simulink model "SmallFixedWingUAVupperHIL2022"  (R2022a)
settings: Solver=FixedStepDiscrete  StartTime=0.0  StopTime=inf  FixedStep=1/150  RelTol=1e-3
model workspace: external: MAT-File (data not in the file)
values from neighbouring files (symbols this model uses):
  env = struct    [InitDatactrl.m]
  uav = struct    [InitDatactrl.m]    (also in InitDatactrldf.m)
  x = x + points(1, i) * k(i) * ft    [bezir_n.m]
undefined symbols (not defined in the file or in its folder): current_a, current_filtered_a, DiscIntNeverNeededParam, remaining, RGBLED_COLOR_ENUM, RGBLED_MODE_ENUM, voltage_filtered_v, voltage_v
libraries: simulink x10, pixhawk_slib_sensors_actuators x6, pixhawk_slib_uORB_RW x5

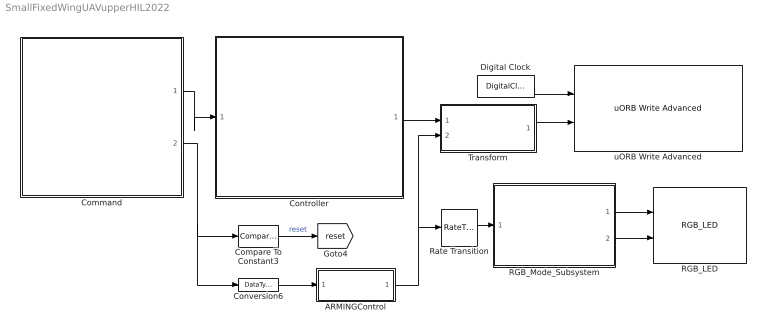
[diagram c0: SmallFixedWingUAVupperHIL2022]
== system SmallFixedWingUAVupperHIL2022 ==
  ARMINGControl : Subsystem
  Command : Subsystem
  Compare To Constant3 : simulink/Logic and Bit Operations/Compare To Constant  relop=<=  const=1100  OutDataTypeStr=boolean
  Controller : Subsystem
  Conversion6 : DataTypeConversion  OutDataTypeStr=double
  Digital Clock : DigitalClock  SampleTime=-1
  RGB_LED : pixhawk_slib_sensors_actuators/RGB_LED
  RGB_Mode_Subsystem : Subsystem
  Rate Transition : RateTransition  OutPortSampleTime=1
  Transform : Subsystem
  uORB Write Advanced : pixhawk_slib_uORB_RW/uORB Write Advanced  Ts=0  uORB_AdvtQueue=on  uORB_FieldEnabledArr="0  0  0  1  0  0  0  0  0  0  0"  uORB_Topic_str=0  uORB_Struct_DT="[1  1  1  1  1]"  BlockInputCount=5  uORB_StructParams="[\"voltage_v\",\"voltage_filtered_v\",\"current_a\",\"current_filtered_a\",\"remaining\"]"  uORB_PortSizes="[1  1  1  1]"  MsgSizeOf=0  MW_update=true
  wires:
  Digital Clock/1 -> uORB Write Advanced/1
  RGB_Mode_Subsystem/1(RGB_MODE) -> RGB_LED/1
  Rate Transition/1 -> RGB_Mode_Subsystem/1(ARM_STATE)
  ARMINGControl/1(Out1) -> Transform/2(Arm), Rate Transition/1
  RGB_Mode_Subsystem/2(RGB_COLOR) -> RGB_LED/2
  Conversion6/1 -> ARMINGControl/1(In1)
  Compare To Constant3/1 -> [reset]  "reset"
  Transform/1(PWMOuput) -> uORB Write Advanced/2
  Controller/1(ActuatorCmd) -> Transform/1(ActuatorCmd)
  Command/2(Arm) -> Conversion6/1, Compare To Constant3/1
  Command/1(Command) -> Controller/1(Cmd)

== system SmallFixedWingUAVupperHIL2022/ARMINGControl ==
  In1 : Inport
  Compare To Constant3 : simulink/Logic and Bit Operations/Compare To Constant  relop=>=  const=uint16(1500)  OutDataTypeStr=boolean
  Out1 : Outport  VectorParamsAs1DForOutWhenUnconnected=off
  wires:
  Compare To Constant3/1 -> Out1/1
  In1/1 -> Compare To Constant3/1

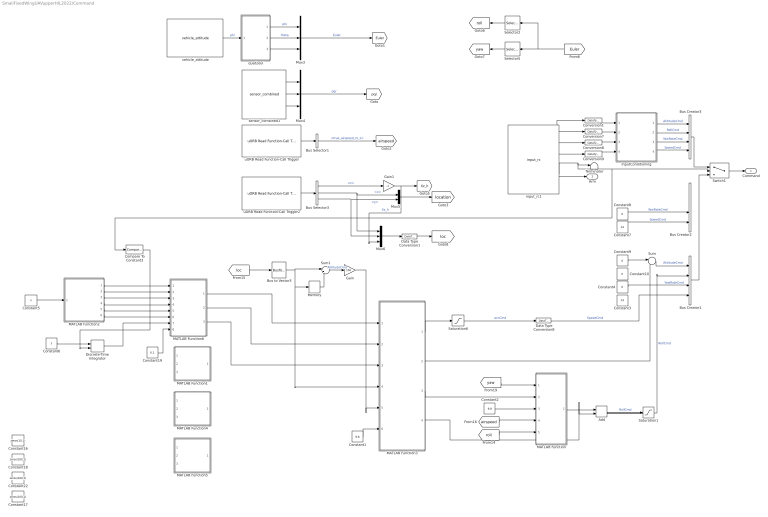
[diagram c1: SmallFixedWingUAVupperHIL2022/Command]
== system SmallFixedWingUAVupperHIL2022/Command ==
  Add : Sum
  Bus Creator1 : BusCreator  Inputs=4
  Bus Creator2 : BusCreator  Inputs=4
  Bus Creator3 : BusCreator  Inputs=4
  Bus Selector1 : BusSelector  OutputSignals=true_airspeed_m_s
  Bus Selector3 : BusSelector  OutputSignals=z,x,y
  Bus to Vector3 : BusToVector
  Compare To Constant3 : simulink/Logic and Bit Operations/Compare To Constant  relop=>=  const=uint16(1500)  OutDataTypeStr=boolean
  Constant1 : Constant  Value=9.8
  Constant{4,8..10} (4 alike) : Constant  Value=0  SampleTime=-1
  Constant16 : Constant  Value=zeros(10,1)
  Constant17 : Constant  Value=zeros(100,1)
  Constant18 : Constant  Value=zeros(100,1)
  Constant19 : Constant  Value=0.1
  Constant2 : Constant  Value=9.8  SampleTime=-1
  Constant22 : Constant  Value=zeros(100,1)
  Constant3 : Constant  Value=14  SampleTime=-1
  Constant5 : Constant  Value=x
  Constant6 : Constant
  Constant7 : Constant  Value=14  SampleTime=-1
  Conversion{1,7..9} (4 alike) : DataTypeConversion  OutDataTypeStr=double
  Data Type Conversion1 : DataTypeConversion  OutDataTypeStr=double
  Data Type Conversion8 : DataTypeConversion  OutDataTypeStr=single
  Discrete-Time Integrator : DiscreteIntegrator  ExternalReset=either  SampleTime=-1  ICPrevOutput=DiscIntNeverNeededParam  ICPrevScaledInput=DiscIntNeverNeededParam
  Gain : Gain  Gain=150
  Gain1 : Gain  Gain=-1
  InputConditioning : Subsystem
  MATLAB Function : MATLAB Function  TreatAsAtomicUnit=on
  MATLAB Function1 : MATLAB Function  Commented=on  TreatAsAtomicUnit=on
  MATLAB Function2 : MATLAB Function  TreatAsAtomicUnit=on
  MATLAB Function3 : MATLAB Function  TreatAsAtomicUnit=on
  MATLAB Function4 : MATLAB Function  Commented=on  TreatAsAtomicUnit=on
  MATLAB Function5 : MATLAB Function  Commented=on  TreatAsAtomicUnit=on
  MATLAB Function6 : MATLAB Function  TreatAsAtomicUnit=on
  Memory : Memory  InheritSampleTime=on
  Mux3 : Mux  Inputs=3
  Mux4 : Mux  Inputs=3
  Mux5 : Mux  Inputs=2
  Mux6 : Mux  Inputs=3
  Saturation1 : Saturate  UpperLimit=0.4  LowerLimit=-0.4
  Saturation6 : Saturate  UpperLimit=10  LowerLimit=-10
  Selector2 : Selector  InputPortWidth=3  IndexOptions=Index vector (dialog)  Indices=1  OutputSizes=1
  Selector5 : Selector  InputPortWidth=3  IndexOptions=Index vector (dialog)  Indices=3  OutputSizes=1
  Sum : Sum  Inputs=|++
  Sum1 : Sum  Inputs=|+-
  Switch1 : Switch  Criteria=u2 > Threshold  Threshold=1500
  Terminator : Terminator
  input_rc1 : pixhawk_slib_sensors_actuators/input_rc  Description=|  sampletime=1/150  channel1=on  channel2=on  channel3=on  channel4=on  channel5=on  channel6=on  channel7=off  channel8=off  channel9=off  channel10=off  channel11=off  channel12=off  channel13=off  channel14=off  channel15=off  channel16=off  channel17=off  channel18=off  ch_count=off  rssi=off  rc_failsafe=off  rc_lost=off  rc_inputsource=off
      | RC Input Block
      | 
      | This block provides user input control to the model.
      | It uses the input_rc uORB topic.
      | 
      | The user has the ability to choose which channels are available as outputs from this block and also some optional outputs. These include 
      | Channels 1 through 18
      | double data type indicating the PWM value from the controller 
      | measured pulse widths for each of the supported channels 
      | Channel Count 
      | u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
  quat2eul : MATLAB Function  TreatAsAtomicUnit=on
  sensor_combined1 : pixhawk_slib_sensors_actuators/sensor_combined  Description=|  sampletime=1/150  show_mag=off  show_acc=off  show_gyro=on  show_baro=off  show_ts=off
      | Sensor Combined Block
      | 
      | This block enables access to the various sensors available on the px4fmu-v2 hardware.  
      | The user can use these signals in the Simulink control model.  
      | The sample time needs to be provided in the mask dialog.  
      | Optional output ports can also be selected.  
      | Refer to the sample model: px4demo_attitude_control.slx
      | 
      | Signal definitions: 
      | Magnetometer (x,y,z) - single values – Mag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
  uORB Read Function-Call Trigger : pixhawk_slib_uORB_RW/uORB Read Function-Call Trigger  uORB_Topic_str='airspeed'  BusObjVar=Bus: airspeed_SL  uORB_Interval=1  AsyncOutput=off  Fcn_call_select=Generate Function Call Signal  TaskName='Task1'  Poll_timeout=100  Ts=-1
  uORB Read Function-Call Trigger2 : pixhawk_slib_uORB_RW/uORB Read Function-Call Trigger  uORB_Topic_str='vehicle_local_position'  BusObjVar=Bus: vehicle_local_position_SL  uORB_Interval=1  AsyncOutput=off  Fcn_call_select=Generate Function Call Signal  TaskName='Task1'  Poll_timeout=100  Ts=-1
  vehicle_attitude : pixhawk_slib_sensors_actuators/vehicle_attitude  sampletime=1/150  show_r=off  show_p=off  show_y=off  show_q=on  show_ts=off
  Command : Outport  VectorParamsAs1DForOutWhenUnconnected=off
  Arm : Outport  Port=2  VectorParamsAs1DForOutWhenUnconnected=off
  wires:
  InputConditioning/3(yawRate_d) -> Bus Creator3/3  "YawRateCmd"
  input_rc1/3 -> Conversion8/1
  input_rc1/2 -> Conversion7/1
  Conversion9/1 -> InputConditioning/4(ch4)
  InputConditioning/2(Roll_d) -> Bus Creator3/2  "RollCmd"
  Constant8/1 -> Bus Creator2/3  "YawRateCmd"
  input_rc1/4 -> Conversion9/1
  InputConditioning/4(Speed_d) -> Bus Creator3/4  "SpeedCmd"
  Conversion1/1 -> InputConditioning/1("ch1 ")
  InputConditioning/1(Altitude_d) -> Bus Creator3/1  "AlititudeCmd"
  input_rc1/5 -> Compare To Constant3/1, Switch1/2, Terminator/1
  Conversion8/1 -> InputConditioning/3(ch3)
  Constant7/1 -> Bus Creator2/4  "SpeedCmd"
  Bus Creator3/1 -> Switch1/1
  input_rc1/1 -> Conversion1/1
  Conversion7/1 -> InputConditioning/2(ch2)
  Switch1/1 -> Command/1
  input_rc1/6 -> Arm/1
  MATLAB Function3/4(roll) -> Add/2
  Saturation6/1 -> Data Type Conversion8/1  "accCmd"
  [airspeed] -> MATLAB Function/4(V)
  MATLAB Function3/3(yaw) -> MATLAB Function/2(yawdes)
  Bus to Vector3/1 -> Sum1/1, Memory/1, MATLAB Function3/4(x)
  Constant2/1 -> MATLAB Function/3(g)
  Constant1/1 -> MATLAB Function3/6(g)
  MATLAB Function/1(roll) -> Add/1
  MATLAB Function3/1(av1) -> Saturation6/1
  [loc] -> Bus to Vector3/1
  [roll] -> MATLAB Function/5(rolldes)
  [yaw] -> MATLAB Function/1(yaw)
  sensor_combined1/3 -> Mux4/3
  Mux4/1 -> [pqr]  "pqr"
  Mux3/1 -> [Euler]  "Euler"
  quat2eul/1(phi) -> Mux3/1  "phi"
  uORB Read Function-Call Trigger/1 -> Bus Selector1/1
  Bus Selector1/1 -> [airspeed]  "<true_airspeed_m_s>"
  vehicle_attitude/1 -> quat2eul/1(q)  "phi"
  quat2eul/2(theta) -> Mux3/2  "theta"
  sensor_combined1/2 -> Mux4/2
  sensor_combined1/1 -> Mux4/1
  quat2eul/3(psi) -> Mux3/3
  Mux6/1 -> Data Type Conversion1/1
  Bus Selector3/2 -> Mux6/1, Mux5/1  "<x>"
  Bus Selector3/3 -> Mux6/2, Mux5/2  "<y>"
  Bus Selector3/1 -> Gain1/1  "<z>"
  Gain1/1 -> Mux6/3, [Xz_h]  "Xz_h"
  Mux5/1 -> [location]
  uORB Read Function-Call Trigger2/1 -> Bus Selector3/1
  Data Type Conversion1/1 -> [loc]
  Selector2/1 -> [roll]
  Selector5/1 -> [yaw]
  [Euler] -> Selector2/1, Selector5/1
  Add/1 -> Saturation1/1  "RollCmd"
  Sum/1 -> Bus Creator1/1  "AlititudeCmd"
  Constant4/1 -> Bus Creator1/3  "YawRateCmd"
  Constant9/1 -> Sum/1
  Data Type Conversion8/1 -> Bus Creator1/4  "SpeedCmd"
  Bus Creator1/1 -> Switch1/3
  Memory/1 -> Sum1/2
  Sum1/1 -> Gain/1  "AlititudeCmd"
  Gain/1 -> MATLAB Function3/5(dx)
  Constant5/1 -> MATLAB Function2/1(x)
  MATLAB Function3/2(Hz) -> Sum/2
  Constant19/1 -> MATLAB Function6/8(sample_tt)
  MATLAB Function2/1(xx) -> MATLAB Function6/1(x)
  MATLAB Function6/1(xdx) -> MATLAB Function3/1(xd)
  MATLAB Function6/2(vdv) -> MATLAB Function3/2(dxd)
  MATLAB Function6/3(ada) -> MATLAB Function3/3(ddxd)
  Constant6/1 -> Discrete-Time Integrator/1
  Discrete-Time Integrator/1 -> MATLAB Function6/7(t)
  MATLAB Function2/2(y) -> MATLAB Function6/2(y)
  MATLAB Function2/3(dx) -> MATLAB Function6/3(dx)
  MATLAB Function2/4(dy) -> MATLAB Function6/4(dy)
  MATLAB Function2/5(ddx) -> MATLAB Function6/5(ddx)
  MATLAB Function2/6(ddy) -> MATLAB Function6/6(ddy)
  Saturation1/1 -> Bus Creator1/2  "RollCmd"
  Compare To Constant3/1 -> Discrete-Time Integrator/2

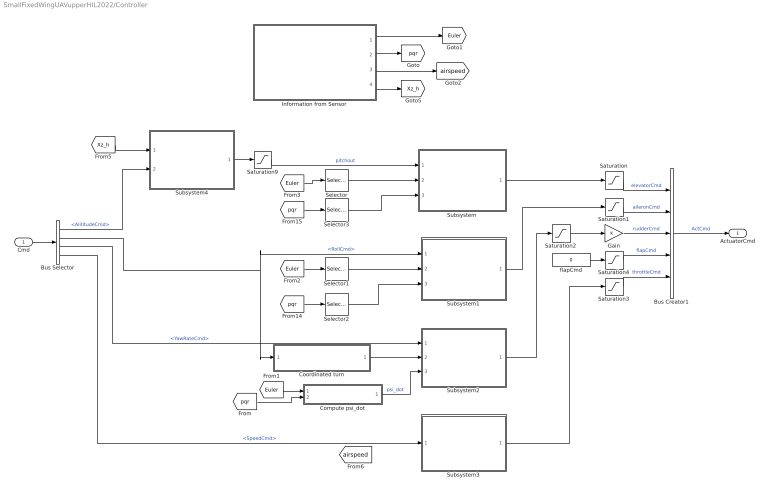
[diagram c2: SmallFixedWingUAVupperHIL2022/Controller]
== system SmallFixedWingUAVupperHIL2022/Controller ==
  Cmd : Inport
  Bus Creator1 : BusCreator  Inputs=5
  Bus Selector : BusSelector  OutputSignals=AlititudeCmd,RollCmd,YawRateCmd,SpeedCmd
  Compute psi_dot : Subsystem
  Coordinated turn : Subsystem
  Gain : Gain
  Information from Sensor : Subsystem
  Saturation : Saturate  UpperLimit=uav.elevator.max  LowerLimit=uav.elevator.min
  Saturation1 : Saturate  UpperLimit=uav.aileron.max  LowerLimit=uav.aileron.min
  Saturation2 : Saturate  UpperLimit=uav.rudder.max  LowerLimit=uav.rudder.min
  Saturation3 : Saturate  UpperLimit=uav.throttlepercent.max  LowerLimit=uav.throttlepercent.min
  Saturation4 : Saturate  UpperLimit=uav.flap.max  LowerLimit=uav.flap.min
  Saturation9 : Saturate  UpperLimit=uav.attitudectrlmax.pitch  LowerLimit=-uav.attitudectrlmax.pitch
  Selector : Selector  InputPortWidth=3  IndexOptions=Index vector (dialog)  Indices=2  OutputSizes=1
  Selector1 : Selector  InputPortWidth=3  IndexOptions=Index vector (dialog)  Indices=1  OutputSizes=1
  Selector2 : Selector  InputPortWidth=3  IndexOptions=Index vector (dialog)  Indices=1  OutputSizes=1
  Selector3 : Selector  InputPortWidth=3  IndexOptions=Index vector (dialog)  Indices=2  OutputSizes=1
  Subsystem : Subsystem
  Subsystem1 : Subsystem
  Subsystem2 : Subsystem
  Subsystem3 : Subsystem
  Subsystem4 : Subsystem
  flapCmd : Constant  Value=0  OutDataTypeStr=double
  ActuatorCmd : Outport  VectorParamsAs1DForOutWhenUnconnected=off
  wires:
  [Euler] -> Selector/1
  Saturation9/1 -> Subsystem/1(pitchout)  "pitchout"
  Selector1/1 -> Subsystem1/2(phi)
  Bus Selector/4 -> Subsystem3/1(<SpeedCmd>)  "<SpeedCmd>"
  Bus Selector/3 -> Subsystem2/1(<YawRateCmd>)  "<YawRateCmd>"
  Bus Selector/1 -> Subsystem4/2(<AlititudeCmd>)  "<AlititudeCmd>"
  Saturation2/1 -> Gain/1
  [pqr] -> Selector2/1
  Subsystem1/1(aileronCmd) -> Saturation1/1
  Information from Sensor/1(Euler) -> [Euler]
  Subsystem2/1(rudderCmd) -> Saturation2/1
  Compute psi_dot/1(psi_dot) -> Subsystem2/3(psi_dot)  "psi_dot"
  Saturation3/1 -> Bus Creator1/5  "throttleCmd"
  Coordinated turn/1(YawRateCmd from Roll) -> Subsystem2/2(In2)
  Selector/1 -> Subsystem/2(theta)
  [Euler] -> Compute psi_dot/1(Euler)
  [Euler] -> Selector1/1
  Subsystem3/1(throttleCmd) -> Saturation3/1
  Bus Selector/2 -> Coordinated turn/1(<RollCmd>), Subsystem1/1(<RollCmd>)  "<RollCmd>"
  [Xz_h] -> Subsystem4/1(In1)
  Selector2/1 -> Subsystem1/3(p)
  Gain/1 -> Bus Creator1/3  "rudderCmd"
  Information from Sensor/3(<true_airspeed_m_s>) -> [airspeed]
  [pqr] -> Selector3/1
  Subsystem4/1(pitchout) -> Saturation9/1
  flapCmd/1 -> Saturation4/1
  [pqr] -> Compute psi_dot/2(G)
  Selector3/1 -> Subsystem/3(q)
  Cmd/1 -> Bus Selector/1
  Information from Sensor/2(pqr) -> [pqr]
  Information from Sensor/4(Xz_h) -> [Xz_h]
  Saturation/1 -> Bus Creator1/1  "elevatorCmd"
  Subsystem/1(elevatorCmd) -> Saturation/1
  Saturation4/1 -> Bus Creator1/4  "flapCmd"
  Saturation1/1 -> Bus Creator1/2  "aileronCmd"
  Bus Creator1/1 -> ActuatorCmd/1  "ActCmd"

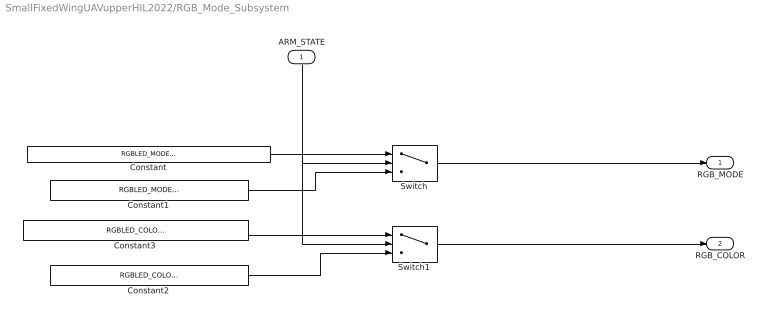
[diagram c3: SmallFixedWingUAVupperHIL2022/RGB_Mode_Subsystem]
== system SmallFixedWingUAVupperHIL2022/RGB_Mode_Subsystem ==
  ARM_STATE : Inport
  Constant : Constant  Value=RGBLED_MODE_ENUM.SL_MODE_BLINK_FAST  OutDataTypeStr=Enum: RGBLED_MODE_ENUM
  Constant1 : Constant  Value=RGBLED_MODE_ENUM.SL_MODE_BREATHE  OutDataTypeStr=Enum: RGBLED_MODE_ENUM
  Constant2 : Constant  Value=RGBLED_COLOR_ENUM.SL_COLOR_GREEN  OutDataTypeStr=Enum: RGBLED_COLOR_ENUM
  Constant3 : Constant  Value=RGBLED_COLOR_ENUM.SL_COLOR_BLUE  OutDataTypeStr=Enum: RGBLED_COLOR_ENUM
  Switch : Switch  Criteria=u2 ~= 0  Threshold=1500
  Switch1 : Switch  Criteria=u2 ~= 0  Threshold=1500
  RGB_MODE : Outport  VectorParamsAs1DForOutWhenUnconnected=off
  RGB_COLOR : Outport  Port=2  VectorParamsAs1DForOutWhenUnconnected=off
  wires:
  ARM_STATE/1 -> Switch1/2, Switch/2
  Constant/1 -> Switch/1
  Constant1/1 -> Switch/3
  Switch/1 -> RGB_MODE/1
  Constant3/1 -> Switch1/1
  Constant2/1 -> Switch1/3
  Switch1/1 -> RGB_COLOR/1

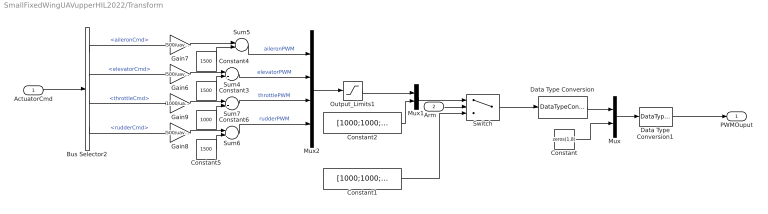
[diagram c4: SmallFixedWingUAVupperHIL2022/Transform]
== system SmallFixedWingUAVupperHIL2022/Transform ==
  ActuatorCmd : Inport
  Arm : Inport  Port=2
  Bus Selector2 : BusSelector  OutputSignals=aileronCmd,elevatorCmd,throttleCmd,rudderCmd
  Constant : Constant  Value=zeros(1,8)
  Constant1 : Constant  Value=[1000;1000;1000;1000;1000;1000;1000;1000]
  Constant2 : Constant  Value=[1000;1000;1000;1000]
  Constant3 : Constant  Value=1500
  Constant4 : Constant  Value=1500
  Constant5 : Constant  Value=1500
  Constant6 : Constant  Value=1000
  Data Type Conversion : DataTypeConversion  OutDataTypeStr=double
  Data Type Conversion1 : DataTypeConversion  OutDataTypeStr=single
  Gain6 : Gain  Gain=500/uav.controlsurfacemax
  Gain7 : Gain  Gain=500/uav.controlsurfacemax
  Gain8 : Gain  Gain=500/uav.controlsurfacemax
  Gain9 : Gain  Gain=1000/uav.throttlepercent.max
  Mux : Mux  Inputs=2
  Mux1 : Mux  Inputs=2
  Mux2 : Mux
  Output_Limits1 : Saturate  UpperLimit=2000  LowerLimit=1000
  Sum{4..7} (4 alike) : Sum  Inputs=|++
  Switch : Switch  Criteria=u2 > Threshold  Threshold=0.5
  PWMOuput : Outport  VectorParamsAs1DForOutWhenUnconnected=off
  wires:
  Constant2/1 -> Mux1/2
  Sum6/1 -> Mux2/4  "rudderPWM"
  Data Type Conversion/1 -> Mux/1
  Bus Selector2/4 -> Gain8/1  "<rudderCmd>"
  Bus Selector2/2 -> Gain6/1  "<elevatorCmd>"
  Constant3/1 -> Sum4/2
  Switch/1 -> Data Type Conversion/1
  Gain6/1 -> Sum4/1
  Bus Selector2/3 -> Gain9/1  "<throttleCmd>"
  Bus Selector2/1 -> Gain7/1  "<aileronCmd>"
  Constant/1 -> Mux/2
  Gain8/1 -> Sum6/1
  Sum7/1 -> Mux2/3  "throttlePWM"
  Constant1/1 -> Switch/3
  Mux1/1 -> Switch/1
  Output_Limits1/1 -> Mux1/1
  Constant5/1 -> Sum6/2
  Sum5/1 -> Mux2/1  "aileronPWM"
  Sum4/1 -> Mux2/2  "elevatorPWM"
  Constant6/1 -> Sum7/2
  Mux2/1 -> Output_Limits1/1
  Gain7/1 -> Sum5/1
  Mux/1 -> Data Type Conversion1/1
  Gain9/1 -> Sum7/1
  Constant4/1 -> Sum5/2
  Arm/1 -> Switch/2
  ActuatorCmd/1 -> Bus Selector2/1
  Data Type Conversion1/1 -> PWMOuput/1

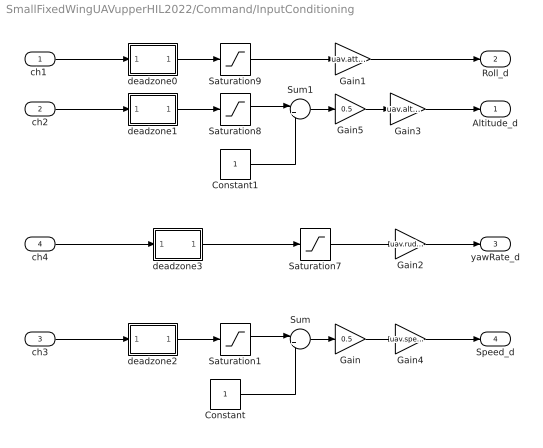
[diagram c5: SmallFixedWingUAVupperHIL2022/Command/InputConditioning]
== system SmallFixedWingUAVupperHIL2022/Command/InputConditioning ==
  "ch1 " : Inport
  ch2 : Inport  Port=2
  ch3 : Inport  Port=3
  ch4 : Inport  Port=4
  Constant : Constant
  Constant1 : Constant
  Gain : Gain  Gain=0.5
  Gain1 : Gain  Gain=uav.attitudectrlmax.roll  OutDataTypeStr=Inherit: Inherit via back propagation
  Gain2 : Gain  Gain=uav.rudder.max
  Gain3 : Gain  Gain=uav.altitude.max  OutDataTypeStr=Inherit: Inherit via back propagation
  Gain4 : Gain  Gain=uav.speed.max
  Gain5 : Gain  Gain=0.5
  Saturation{1,7..9} (4 alike) : Saturate  UpperLimit=1  LowerLimit=-1
  Sum : Sum  Inputs=|++
  Sum1 : Sum  Inputs=|++
  deadzone0 : MATLAB Function  TreatAsAtomicUnit=on
  deadzone1 : MATLAB Function  TreatAsAtomicUnit=on
  deadzone2 : MATLAB Function  TreatAsAtomicUnit=on
  deadzone3 : MATLAB Function  TreatAsAtomicUnit=on
  Altitude_d : Outport  VectorParamsAs1DForOutWhenUnconnected=off
  Roll_d : Outport  Port=2  VectorParamsAs1DForOutWhenUnconnected=off
  yawRate_d : Outport  Port=3  VectorParamsAs1DForOutWhenUnconnected=off
  Speed_d : Outport  Port=4  VectorParamsAs1DForOutWhenUnconnected=off
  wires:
  deadzone2/1(y) -> Saturation1/1
  ch3/1 -> deadzone2/1(u)
  deadzone1/1(y) -> Saturation8/1
  Gain/1 -> Gain4/1
  deadzone0/1(y) -> Saturation9/1
  "ch1 "/1 -> deadzone0/1(u)
  ch2/1 -> deadzone1/1(u)
  Saturation9/1 -> Gain1/1
  Saturation8/1 -> Sum1/1
  Constant/1 -> Sum/2
  Sum/1 -> Gain/1
  Gain1/1 -> Roll_d/1
  Gain3/1 -> Altitude_d/1
  Saturation7/1 -> Gain2/1
  deadzone3/1(y) -> Saturation7/1
  ch4/1 -> deadzone3/1(u)
  Gain2/1 -> yawRate_d/1
  Saturation1/1 -> Sum/1
  Gain4/1 -> Speed_d/1
  Gain5/1 -> Gain3/1
  Constant1/1 -> Sum1/2
  Sum1/1 -> Gain5/1

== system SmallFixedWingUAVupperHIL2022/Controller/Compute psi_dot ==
  Euler : Inport
  G : Inport  Port=2
  Mux1 : Mux  Inputs=2
  psidot : Fcn  Expr=(u[5]*sin(u[1])+u[6]*cos(u[1]))/cos(u[2])
  psi_dot : Outport  Unit=rad/S  VectorParamsAs1DForOutWhenUnconnected=off
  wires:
  G/1 -> Mux1/2
  psidot/1 -> psi_dot/1  "psi_dot"
  Mux1/1 -> psidot/1
  Euler/1 -> Mux1/1

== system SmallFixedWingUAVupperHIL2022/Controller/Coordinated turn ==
  <RollCmd> : Inport
  Divide : Product  Inputs=*/*
  Trigonometric Function : Trigonometry  Operator=tan
  env.ISA_g : Constant  Value=env.ISA_g
  YawRateCmd from Roll : Outport  VectorParamsAs1DForOutWhenUnconnected=off
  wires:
  env.ISA_g/1 -> Divide/3
  [airspeed] -> Divide/2
  Trigonometric Function/1 -> Divide/1
  Divide/1 -> YawRateCmd from Roll/1  "YawRateCmd from Roll"
  <RollCmd>/1 -> Trigonometric Function/1

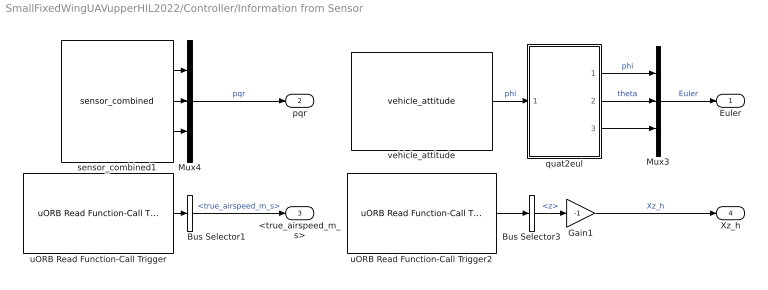
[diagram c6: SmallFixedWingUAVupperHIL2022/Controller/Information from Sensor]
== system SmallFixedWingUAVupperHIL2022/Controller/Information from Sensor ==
  Bus Selector1 : BusSelector  OutputSignals=true_airspeed_m_s
  Bus Selector3 : BusSelector  OutputSignals=z
  Gain1 : Gain  Gain=-1
  Mux3 : Mux  Inputs=3
  Mux4 : Mux  Inputs=3
  quat2eul : MATLAB Function  TreatAsAtomicUnit=on
  sensor_combined1 : pixhawk_slib_sensors_actuators/sensor_combined  Description=|  sampletime=1/150  show_mag=off  show_acc=off  show_gyro=on  show_baro=off  show_ts=off
      | Sensor Combined Block
      | 
      | This block enables access to the various sensors available on the px4fmu-v2 hardware.  
      | The user can use these signals in the Simulink control model.  
      | The sample time needs to be provided in the mask dialog.  
      | Optional output ports can also be selected.  
      | Refer to the sample model: px4demo_attitude_control.slx
      | 
      | Signal definitions: 
      | Magnetometer (x,y,z) - single values – Mag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
  uORB Read Function-Call Trigger : pixhawk_slib_uORB_RW/uORB Read Function-Call Trigger  uORB_Topic_str='airspeed'  BusObjVar=Bus: airspeed_SL  uORB_Interval=1  AsyncOutput=off  Fcn_call_select=Generate Function Call Signal  TaskName='Task1'  Poll_timeout=100  Ts=-1
  uORB Read Function-Call Trigger2 : pixhawk_slib_uORB_RW/uORB Read Function-Call Trigger  uORB_Topic_str='vehicle_local_position'  BusObjVar=Bus: vehicle_local_position_SL  uORB_Interval=1  AsyncOutput=off  Fcn_call_select=Generate Function Call Signal  TaskName='Task1'  Poll_timeout=100  Ts=-1
  vehicle_attitude : pixhawk_slib_sensors_actuators/vehicle_attitude  sampletime=1/150  show_r=off  show_p=off  show_y=off  show_q=on  show_ts=off
  Euler : Outport  VectorParamsAs1DForOutWhenUnconnected=off
  pqr : Outport  Port=2  VectorParamsAs1DForOutWhenUnconnected=off
  <true_airspeed_m_s> : Outport  Port=3  VectorParamsAs1DForOutWhenUnconnected=off
  Xz_h : Outport  Port=4  VectorParamsAs1DForOutWhenUnconnected=off
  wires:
  sensor_combined1/2 -> Mux4/2
  Mux4/1 -> pqr/1  "pqr"
  Mux3/1 -> Euler/1  "Euler"
  Gain1/1 -> Xz_h/1  "Xz_h"
  Bus Selector1/1 -> <true_airspeed_m_s>/1  "<true_airspeed_m_s>"
  quat2eul/3(psi) -> Mux3/3
  quat2eul/1(phi) -> Mux3/1  "phi"
  vehicle_attitude/1 -> quat2eul/1(q)  "phi"
  uORB Read Function-Call Trigger/1 -> Bus Selector1/1
  uORB Read Function-Call Trigger2/1 -> Bus Selector3/1
  sensor_combined1/3 -> Mux4/3
  sensor_combined1/1 -> Mux4/1
  Bus Selector3/1 -> Gain1/1  "<z>"
  quat2eul/2(theta) -> Mux3/2  "theta"

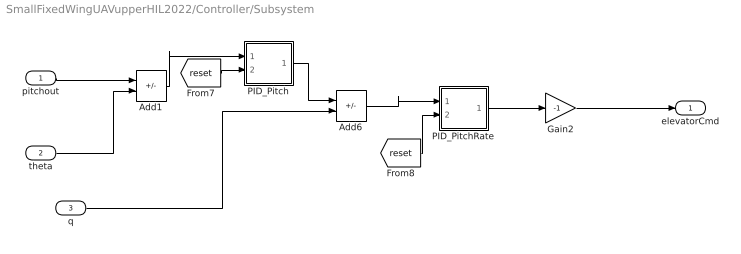
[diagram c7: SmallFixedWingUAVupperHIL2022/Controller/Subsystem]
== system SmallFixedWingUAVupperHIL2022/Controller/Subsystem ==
  pitchout : Inport
  theta : Inport  Port=2
  q : Inport  Port=3
  Add1 : Sum  Inputs=+-
  Add6 : Sum  Inputs=+-
  Gain2 : Gain  Gain=-1
  PID_Pitch : Subsystem
  PID_PitchRate : Subsystem
  elevatorCmd : Outport  VectorParamsAs1DForOutWhenUnconnected=off
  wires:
  PID_PitchRate/1(y) -> Gain2/1
  q/1 -> Add6/2
  Add1/1 -> PID_Pitch/1(x)
  [reset] -> PID_PitchRate/2(reset_i)
  [reset] -> PID_Pitch/2(reset_i)
  theta/1 -> Add1/2
  PID_Pitch/1(y) -> Add6/1
  Add6/1 -> PID_PitchRate/1(x)
  Gain2/1 -> elevatorCmd/1
  pitchout/1 -> Add1/1

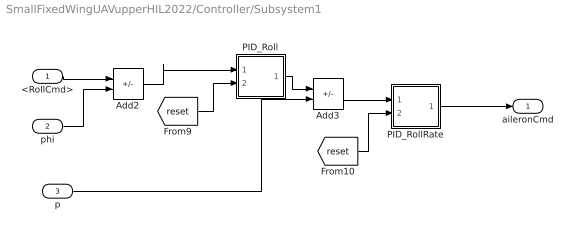
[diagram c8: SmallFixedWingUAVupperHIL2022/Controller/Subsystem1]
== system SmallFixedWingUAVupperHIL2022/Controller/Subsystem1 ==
  <RollCmd> : Inport
  phi : Inport  Port=2
  p : Inport  Port=3
  Add2 : Sum  Inputs=+-
  Add3 : Sum  Inputs=+-
  PID_Roll : Subsystem
  PID_RollRate : Subsystem
  aileronCmd : Outport  VectorParamsAs1DForOutWhenUnconnected=off
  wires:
  Add3/1 -> PID_RollRate/1(x)
  [reset] -> PID_Roll/2(reset_i)
  PID_Roll/1(y) -> Add3/1
  Add2/1 -> PID_Roll/1(x)
  [reset] -> PID_RollRate/2(reset_i)
  PID_RollRate/1(y) -> aileronCmd/1
  phi/1 -> Add2/2
  p/1 -> Add3/2
  <RollCmd>/1 -> Add2/1

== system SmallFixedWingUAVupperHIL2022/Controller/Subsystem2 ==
  <YawRateCmd> : Inport
  In2 : Inport  Port=2
  psi_dot : Inport  Port=3
  Add4 : Sum  Inputs=+-
  PID_YawRate : Subsystem
  Sum2 : Sum  Inputs=++|
  rudderCmd : Outport  VectorParamsAs1DForOutWhenUnconnected=off
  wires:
  Add4/1 -> PID_YawRate/1(x)
  [reset] -> PID_YawRate/2(reset_i)
  psi_dot/1 -> Add4/2
  PID_YawRate/1(y) -> Sum2/2
  <YawRateCmd>/1 -> Sum2/1
  Sum2/1 -> rudderCmd/1
  In2/1 -> Add4/1

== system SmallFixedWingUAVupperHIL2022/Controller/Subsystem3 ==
  <SpeedCmd> : Inport
  Add7 : Sum  Inputs=+-
  PID_Speed : Subsystem
  throttleCmd : Outport  VectorParamsAs1DForOutWhenUnconnected=off
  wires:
  [reset] -> PID_Speed/2(reset_i)
  Add7/1 -> PID_Speed/1(x)  "speederror"
  <SpeedCmd>/1 -> throttleCmd/1

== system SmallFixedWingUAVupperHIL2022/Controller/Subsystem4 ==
  In1 : Inport
  <AlititudeCmd> : Inport  Port=2
  Add8 : Sum  Inputs=+-
  PID_Altitude : Subsystem
  pitchout : Outport  VectorParamsAs1DForOutWhenUnconnected=off
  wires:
  [reset] -> PID_Altitude/2(reset_i)
  In1/1 -> Add8/2
  Add8/1 -> PID_Altitude/1(x)
  <AlititudeCmd>/1 -> Add8/1
  PID_Altitude/1(y) -> pitchout/1  "pitchout"

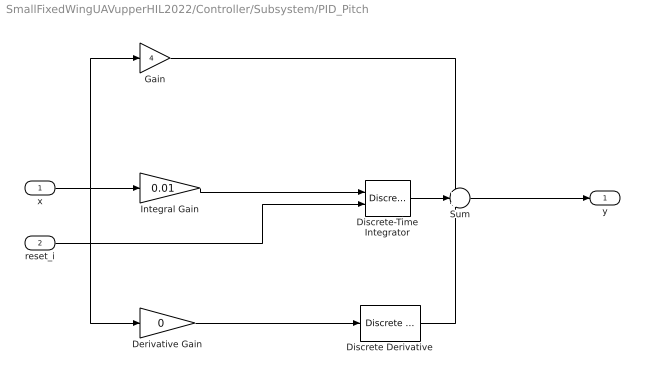
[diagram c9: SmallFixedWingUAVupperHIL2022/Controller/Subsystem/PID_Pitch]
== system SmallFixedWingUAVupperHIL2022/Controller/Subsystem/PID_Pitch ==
  x : Inport
  reset_i : Inport  Port=2
  Derivative Gain : Gain  DisableCoverage=on  Gain=0  ParamMin=-100  ParamMax=100  OutMin=-100  OutMax=100
  Discrete Derivative : simulink/Discrete/Discrete Derivative  gainval=1.0  ICPrevScaledInput=0.0  OutMin=[]  OutMax=[]  OutDataType=fixdt(1, 16)  OutScaling=2^-10  DoSatur=off
  Discrete-Time Integrator : DiscreteIntegrator  ExternalReset=either  SampleTime=-1  ICPrevOutput=DiscIntNeverNeededParam  ICPrevScaledInput=DiscIntNeverNeededParam
  Gain : Gain  Gain=4
  Integral Gain : Gain  DisableCoverage=on  Gain=0.01
  Sum : Sum  Inputs=+++
  y : Outport  InitialOutput=0  VectorParamsAs1DForOutWhenUnconnected=off
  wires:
  reset_i/1 -> Discrete-Time Integrator/2
  Discrete-Time Integrator/1 -> Sum/2
  Discrete Derivative/1 -> Sum/3
  Sum/1 -> y/1
  Gain/1 -> Sum/1
  Derivative Gain/1 -> Discrete Derivative/1
  Integral Gain/1 -> Discrete-Time Integrator/1
  x/1 -> Derivative Gain/1, Integral Gain/1, Gain/1

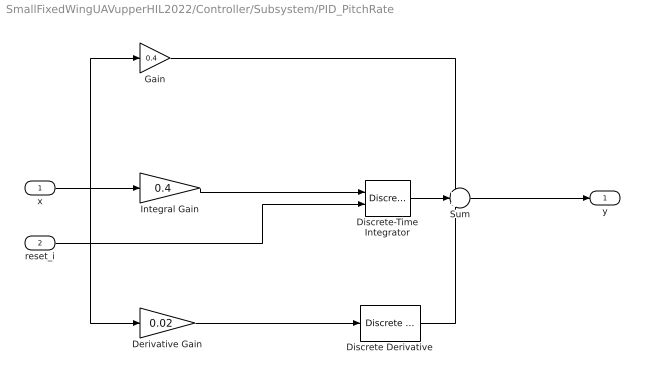
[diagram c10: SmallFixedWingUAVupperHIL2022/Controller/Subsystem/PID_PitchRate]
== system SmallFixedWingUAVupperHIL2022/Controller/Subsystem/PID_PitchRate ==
  x : Inport
  reset_i : Inport  Port=2
  Derivative Gain : Gain  DisableCoverage=on  Gain=0.02  ParamMin=-100  ParamMax=100  OutMin=-100  OutMax=100
  Discrete Derivative : simulink/Discrete/Discrete Derivative  gainval=1.0  ICPrevScaledInput=0.0  OutMin=[]  OutMax=[]  OutDataType=fixdt(1, 16)  OutScaling=2^-10  DoSatur=off
  Discrete-Time Integrator : DiscreteIntegrator  ExternalReset=either  SampleTime=-1  LimitOutput=on  UpperSaturationLimit=0.3  LowerSaturationLimit=-0.3  ICPrevOutput=DiscIntNeverNeededParam  ICPrevScaledInput=DiscIntNeverNeededParam
  Gain : Gain  Gain=0.4
  Integral Gain : Gain  DisableCoverage=on  Gain=0.4
  Sum : Sum  Inputs=+++
  y : Outport  InitialOutput=0  VectorParamsAs1DForOutWhenUnconnected=off
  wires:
  x/1 -> Gain/1, Integral Gain/1, Derivative Gain/1
  Integral Gain/1 -> Discrete-Time Integrator/1
  Derivative Gain/1 -> Discrete Derivative/1
  Gain/1 -> Sum/1
  Sum/1 -> y/1
  Discrete Derivative/1 -> Sum/3
  Discrete-Time Integrator/1 -> Sum/2
  reset_i/1 -> Discrete-Time Integrator/2

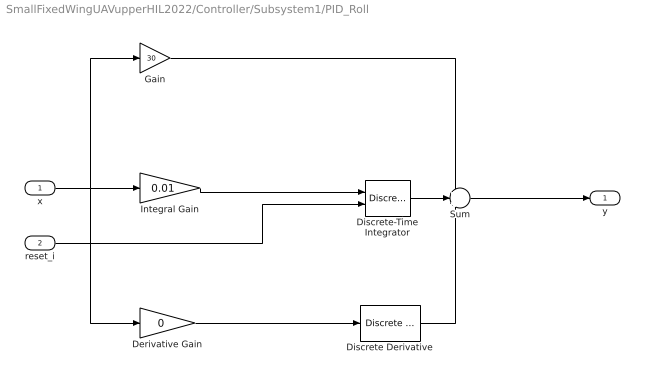
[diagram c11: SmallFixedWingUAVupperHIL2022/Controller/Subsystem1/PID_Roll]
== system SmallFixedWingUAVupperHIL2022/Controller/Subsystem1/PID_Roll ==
  x : Inport
  reset_i : Inport  Port=2
  Derivative Gain : Gain  DisableCoverage=on  Gain=0  ParamMin=-100  ParamMax=100  OutMin=-100  OutMax=100
  Discrete Derivative : simulink/Discrete/Discrete Derivative  gainval=1.0  ICPrevScaledInput=0.0  OutMin=[]  OutMax=[]  OutDataType=fixdt(1, 16)  OutScaling=2^-10  DoSatur=off
  Discrete-Time Integrator : DiscreteIntegrator  ExternalReset=either  SampleTime=-1  ICPrevOutput=DiscIntNeverNeededParam  ICPrevScaledInput=DiscIntNeverNeededParam
  Gain : Gain  Gain=30
  Integral Gain : Gain  DisableCoverage=on  Gain=0.01
  Sum : Sum  Inputs=+++
  y : Outport  InitialOutput=0  VectorParamsAs1DForOutWhenUnconnected=off
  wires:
  x/1 -> Gain/1, Integral Gain/1, Derivative Gain/1
  Integral Gain/1 -> Discrete-Time Integrator/1
  Derivative Gain/1 -> Discrete Derivative/1
  Gain/1 -> Sum/1
  Sum/1 -> y/1
  Discrete Derivative/1 -> Sum/3
  Discrete-Time Integrator/1 -> Sum/2
  reset_i/1 -> Discrete-Time Integrator/2

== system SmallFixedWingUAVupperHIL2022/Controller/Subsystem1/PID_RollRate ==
  x : Inport
  reset_i : Inport  Port=2
  Derivative Gain : Gain  DisableCoverage=on  Gain=0.05  ParamMin=-100  ParamMax=100  OutMin=-100  OutMax=100
  Discrete Derivative : simulink/Discrete/Discrete Derivative  gainval=1.0  ICPrevScaledInput=0.0  OutMin=[]  OutMax=[]  OutDataType=fixdt(1, 16)  OutScaling=2^-10  DoSatur=off
  Discrete-Time Integrator : DiscreteIntegrator  ExternalReset=either  SampleTime=-1  LimitOutput=on  UpperSaturationLimit=0.3  LowerSaturationLimit=-0.3  ICPrevOutput=DiscIntNeverNeededParam  ICPrevScaledInput=DiscIntNeverNeededParam
  Gain : Gain
  Integral Gain : Gain  DisableCoverage=on  Gain=0.6
  Sum : Sum  Inputs=+++
  y : Outport  InitialOutput=0  VectorParamsAs1DForOutWhenUnconnected=off
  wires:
  reset_i/1 -> Discrete-Time Integrator/2
  Discrete-Time Integrator/1 -> Sum/2
  Discrete Derivative/1 -> Sum/3
  Sum/1 -> y/1
  Gain/1 -> Sum/1
  Derivative Gain/1 -> Discrete Derivative/1
  Integral Gain/1 -> Discrete-Time Integrator/1
  x/1 -> Derivative Gain/1, Integral Gain/1, Gain/1

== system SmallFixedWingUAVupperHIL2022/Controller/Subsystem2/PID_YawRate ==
  x : Inport
  reset_i : Inport  Port=2
  Derivative Gain : Gain  DisableCoverage=on  Gain=0.01  ParamMin=-100  ParamMax=100  OutMin=-100  OutMax=100
  Discrete Derivative : simulink/Discrete/Discrete Derivative  gainval=1.0  ICPrevScaledInput=0.0  OutMin=[]  OutMax=[]  OutDataType=fixdt(1, 16)  OutScaling=2^-10  DoSatur=off
  Discrete-Time Integrator : DiscreteIntegrator  ExternalReset=either  SampleTime=-1  LimitOutput=on  UpperSaturationLimit=0.3  LowerSaturationLimit=-0.3  ICPrevOutput=DiscIntNeverNeededParam  ICPrevScaledInput=DiscIntNeverNeededParam
  Gain : Gain  Gain=1.2
  Integral Gain : Gain  DisableCoverage=on  Gain=0.2
  Sum : Sum  Inputs=+++
  y : Outport  InitialOutput=0  VectorParamsAs1DForOutWhenUnconnected=off
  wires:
  x/1 -> Gain/1, Integral Gain/1, Derivative Gain/1
  Integral Gain/1 -> Discrete-Time Integrator/1
  Derivative Gain/1 -> Discrete Derivative/1
  Gain/1 -> Sum/1
  Sum/1 -> y/1
  Discrete Derivative/1 -> Sum/3
  Discrete-Time Integrator/1 -> Sum/2
  reset_i/1 -> Discrete-Time Integrator/2

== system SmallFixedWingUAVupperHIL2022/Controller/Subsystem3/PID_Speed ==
  x : Inport
  reset_i : Inport  Port=2
  Derivative Gain : Gain  DisableCoverage=on  Gain=0  ParamMin=-100  ParamMax=100  OutMin=-100  OutMax=100
  Discrete Derivative : simulink/Discrete/Discrete Derivative  gainval=1.0  ICPrevScaledInput=0.0  OutMin=[]  OutMax=[]  OutDataType=fixdt(1, 16)  OutScaling=2^-10  DoSatur=off
  Discrete-Time Integrator : DiscreteIntegrator  ExternalReset=either  SampleTime=-1  UpperSaturationLimit=0.3  LowerSaturationLimit=-0.3  ICPrevOutput=DiscIntNeverNeededParam  ICPrevScaledInput=DiscIntNeverNeededParam
  Gain : Gain
  Integral Gain : Gain  DisableCoverage=on  Gain=0
  Sum : Sum  Inputs=+++
  y : Outport  InitialOutput=0  VectorParamsAs1DForOutWhenUnconnected=off
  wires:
  reset_i/1 -> Discrete-Time Integrator/2
  Discrete-Time Integrator/1 -> Sum/2
  Discrete Derivative/1 -> Sum/3
  Sum/1 -> y/1
  Gain/1 -> Sum/1
  Derivative Gain/1 -> Discrete Derivative/1
  Integral Gain/1 -> Discrete-Time Integrator/1
  x/1 -> Derivative Gain/1, Integral Gain/1, Gain/1

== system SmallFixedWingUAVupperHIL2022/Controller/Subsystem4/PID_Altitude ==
  x : Inport
  reset_i : Inport  Port=2
  Derivative Gain : Gain  DisableCoverage=on  Gain=0  ParamMin=-100  ParamMax=100  OutMin=-100  OutMax=100
  Discrete Derivative : simulink/Discrete/Discrete Derivative  gainval=1.0  ICPrevScaledInput=0.0  OutMin=[]  OutMax=[]  OutDataType=fixdt(1, 16)  OutScaling=2^-10  DoSatur=off
  Discrete-Time Integrator : DiscreteIntegrator  ExternalReset=either  SampleTime=-1  ICPrevOutput=DiscIntNeverNeededParam  ICPrevScaledInput=DiscIntNeverNeededParam
  Gain : Gain  Gain=0.05
  Integral Gain : Gain  DisableCoverage=on  Gain=0
  Sum : Sum  Inputs=+++
  y : Outport  InitialOutput=0  VectorParamsAs1DForOutWhenUnconnected=off
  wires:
  x/1 -> Gain/1, Integral Gain/1, Derivative Gain/1
  Integral Gain/1 -> Discrete-Time Integrator/1
  Derivative Gain/1 -> Discrete Derivative/1
  Gain/1 -> Sum/1
  Sum/1 -> y/1
  Discrete Derivative/1 -> Sum/3
  Discrete-Time Integrator/1 -> Sum/2
  reset_i/1 -> Discrete-Time Integrator/2

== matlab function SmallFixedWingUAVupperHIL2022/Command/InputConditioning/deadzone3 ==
function y = fcn(u)
%Function description:
%  Control the range of the remote control input from RCMin to RCMax, and set
%  a dead zone with a dead zone size of ±deadZone,the output y is
%  normalized to 0~1.You can get the RC calibration parameters in QGC.
RCMin = 1100;
RCMax = 1900;
RCMid = (RCMin + RCMax)/2;
deadZoneRate = 0.05;
deadZone = deadZoneRate*(RCMax - RCMin);
k = 1/(RCMax - RCMid - deadZone);
%Limiting
if(u < RCMin)
    u = RCMin;
elseif(u > RCMax)
    u = RCMax;
end
%dead zone and normalize
 if(u > RCMid + deadZone)
    y = (u-RCMid - deadZone)*k;
 elseif(u < RCMid - deadZone)
     y = (u - RCMid + deadZone)*k;
 else
     y = 0;
 end

 end

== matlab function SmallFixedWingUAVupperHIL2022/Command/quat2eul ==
function [phi,theta,psi] = quat2eul(q)
% Conversion from Quaternion to Euler angles based on the PX4 Firmware
% v1.6.5 release.
% 
% Quaternion -> DCM -> Euler Angles
% INPUT:
%   q: Quaternion vector of the format: (a + bi + cj + dk)
% OUTPUT:
%   [phi,theta,psi]: Euler angles in radians.
% 
 
    a = q(1);
    b = q(2);
    c = q(3);
    d = q(4);

    aSq = a*a;
    bSq = b*b;
    cSq = c*c;
    dSq = d*d;

    d_pi2 = pi/2;

    % quaternion_to_dcm
    dcm00 = aSq + bSq - cSq - dSq;
    % dcm01 = 2*(b*c - a*d);
    dcm02 = 2*(a*c + b*d);
    dcm10 = 2*(b*c + a*d);
    % dcm11 = aSq - bSq + cSq - dSq;
    dcm12 = 2*(c*d - a*b);
    dcm20 = 2*(b*d - a*c);
    dcm21 = 2*(a*b + c*d);
    dcm22 = aSq - bSq - cSq + dSq;

    % dcm_to_euler
    theta = asin(-dcm20);
    if abs(theta - d_pi2) < 1.0e-3
        phi = single(0.0);
        psi = atan2(dcm12, dcm02);
    elseif abs(theta + d_pi2) < 1.0e-3
        phi = single(0.0);
        psi = atan2(-dcm12, -dcm02);
    else
        phi = atan2(dcm21, dcm22);
        psi = atan2(dcm10, dcm00);
    end

end

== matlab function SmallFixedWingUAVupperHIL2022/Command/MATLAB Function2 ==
function [xx,y,dx,dy,ddx,ddy]  = track(x)
%     index = int8(t/sample_tt);
%     if index <= 1
%         index = int8(1);
%     end
%     if index >= length(x)
%         index = int8(length(x));
%     end
    len = length(x)/6;

    xx = x(1:len);
    y = x(len+1:2*len);
    dx = x(2*len+1:3*len);
    dy = x(3*len+1:4*len);
    ddx = x(4*len+1:5*len);
    ddy = x(5*len+1:6*len);
end

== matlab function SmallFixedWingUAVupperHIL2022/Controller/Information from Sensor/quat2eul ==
function [phi,theta,psi] = quat2eul(q)
% Conversion from Quaternion to Euler angles based on the PX4 Firmware
% v1.6.5 release.
% 
% Quaternion -> DCM -> Euler Angles
% INPUT:
%   q: Quaternion vector of the format: (a + bi + cj + dk)
% OUTPUT:
%   [phi,theta,psi]: Euler angles in radians.
% 
 
    a = q(1);
    b = q(2);
    c = q(3);
    d = q(4);

    aSq = a*a;
    bSq = b*b;
    cSq = c*c;
    dSq = d*d;

    d_pi2 = pi/2;

    % quaternion_to_dcm
    dcm00 = aSq + bSq - cSq - dSq;
    % dcm01 = 2*(b*c - a*d);
    dcm02 = 2*(a*c + b*d);
    dcm10 = 2*(b*c + a*d);
    % dcm11 = aSq - bSq + cSq - dSq;
    dcm12 = 2*(c*d - a*b);
    dcm20 = 2*(b*d - a*c);
    dcm21 = 2*(a*b + c*d);
    dcm22 = aSq - bSq - cSq + dSq;

    % dcm_to_euler
    theta = asin(-dcm20);
    if abs(theta - d_pi2) < 1.0e-3
        phi = single(0.0);
        psi = atan2(dcm12, dcm02);
    elseif abs(theta + d_pi2) < 1.0e-3
        phi = single(0.0);
        psi = atan2(-dcm12, -dcm02);
    else
        phi = atan2(dcm21, dcm22);
        psi = atan2(dcm10, dcm00);
    end

end

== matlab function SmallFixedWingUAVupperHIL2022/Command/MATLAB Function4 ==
function vdv  = track(x,t,sample_tt)
%     index = int8(t/sample_tt);
%     if index <= 1
%         index = int8(1);
%     end
%     if index >= length(x)
%         index = int8(length(x));
%     end
    index = 1;
    dxx = x(index+300);
    dyy = x(index+400);

    vdv = [dxx;-dyy;0];
end

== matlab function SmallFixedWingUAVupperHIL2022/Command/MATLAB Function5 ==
function ada  = track(x,t,sample_tt)
%     index = int8(t/sample_tt);
%     if index <= 1
%         index = int8(1);
%     end
%     if index >= length(x)
%         index = int8(length(x));
%     end
    index = 10;
    ddxx = x(index+500);
    ddyy = x(index+600);

    ada = [ddxx;-ddyy;0];
end

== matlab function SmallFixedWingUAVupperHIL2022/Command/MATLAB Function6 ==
function [xdx,vdv,ada]  = track(x,y,dx,dy,ddx,ddy,t,sample_tt)
    index = int16(t/sample_tt);
    if index <= 1
        index = int16(1);
    end
    if index >= length(x)
        index = int16(length(x));
    end
    xx = x(index);
    yy = y(index);
    dxx = dx(index);
    dyy = dy(index);
    ddxx = ddx(index);
    ddyy = ddy(index);

    xdx = [xx;-yy;0];
    vdv = [dxx;-dyy;0];
    ada = [ddxx;-ddyy;0];
end

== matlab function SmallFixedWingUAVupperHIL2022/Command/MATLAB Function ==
function roll = fcn(yaw,yawdes,g,V,rolldes)
%     roll = yawrate*g*V;
    if yaw>pi
        yaw = yaw-2*pi;
    end
    yawrate = 2*(yawdes-yaw);
    roll = atan2(V.*yawrate,g);
end

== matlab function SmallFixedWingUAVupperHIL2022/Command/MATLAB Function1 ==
function xdx  = track(x,t,sample_tt)
%     index = int8(t/sample_tt);
%     if index <= 1
%         index = int8(1);
%     end
%     if index >= length(x)
%         index = int8(length(x));
%     end
    index = 1;
    xx = x(index+100);
    yy = x(index+200);

    xdx = [xx;-yy;0];
end

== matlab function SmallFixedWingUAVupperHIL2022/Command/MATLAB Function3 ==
function [av1,Hz,yaw,roll] = DF(xd,dxd,ddxd,x,dx,g)
    av1 = (0); 
    Hz= (0); 
    yaw= (0); 
    roll= (0); 
    xd = [xd(1);xd(2);xd(3)];
    dxd = [dxd(1);dxd(2);dxd(3)];
    ddxd = [ddxd(1);ddxd(2);ddxd(3)];
    x = [x(1);x(2);x(3)];
    dx = [dx(1);dx(2);dx(3)];
%     x1 = (xd-x)/norm(xd-x);
    r1 = zeros(3,1);
    r1 = (dxd+0.2*(xd-x))/(norm(dxd+0.2*(xd-x))+0.001);
    


    av1 = ( r1'*(1*ddxd-[0;0;g]+5*(dxd-dx)+3*(xd-x)));
     %%
%     t1 = zeros(3,1,'single');
%     t2 = zeros(3,1,'single');
%     t3 = zeros(3,1,'single');
%     t4 = zeros(3,1,'single');
%     t1(1,1) = ddxd(1,1);
%     t1(2,1) = ddxd(2,1);
%     t1(3,1) = ddxd(3,1) - single(g);
%     
%     for i = 1:3
%     t2(i,1) = single(3) * (dxd(i,1) - dx(i,1));
%     t3(i,1) = single(0.1) * (xd(i,1) - x(i,1));
% 
%     end
% 
%     for i = 1:3
%     t4(i,1) = t1(i,1) + t2(i,1) + t3(i,1);
%     end
%     av1 = single( r1'*t4);
%%

    an = (eye(3)-(r1*r1'))*((ddxd)-([0;0;g]));

    av3 = -(norm(an));
    
    Hz = (xd(3));


    r3 = (an)/((av3)+(0.001));

    r2 = cross(r3,r1);

    yaw = (atan2(r1(2),r1(1)));
    
    roll = (atan2(r2(3),r3(3)));

    if isnan(av1)
        av1=(0);
    end
    if isnan(Hz)
        Hz=(0);
    end
    if isnan(yaw)
        yaw=(0);
    end

end

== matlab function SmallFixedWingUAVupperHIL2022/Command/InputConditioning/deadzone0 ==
function y = fcn(u)
%Function description:
%  Control the range of the remote control input from RCMin to RCMax,which can be obtained from QGC. And set
%  a dead zone with a dead zone size of deadZone,the output y is normalized to 0~1.
RCMin = 1100;
RCMax = 1900;
RCMid = (RCMin + RCMax)/2;
deadZoneRate = 0.05;
deadZone = deadZoneRate*(RCMax - RCMin);
k = 1/(RCMax - RCMid - deadZone);
%Limiting
if(u < RCMin)
    u = RCMin;
elseif(u > RCMax)
    u = RCMax;
end
%dead zone and normalize
 if(u > RCMid + deadZone)
    y = (u-RCMid - deadZone)*k;
 elseif(u < RCMid - deadZone)
     y = (u - RCMid + deadZone)*k;
 else
     y = 0;
 end

 end

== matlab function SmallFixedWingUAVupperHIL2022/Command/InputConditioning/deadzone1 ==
function y = fcn(u)
%Function description:
%  Control the range of the remote control input from RCMin to RCMax, and set
%  a dead zone with a dead zone size of ±deadZone,the output y is
%  normalized to 0~1.You can get the RC calibration parameters in QGC.
RCMin = 1100;
RCMax = 1900;
RCMid = (RCMin + RCMax)/2;
deadZoneRate = 0.05;
deadZone = deadZoneRate*(RCMax - RCMin);
k = 1/(RCMax - RCMid - deadZone);
%Limiting
if(u < RCMin)
    u = RCMin;
elseif(u > RCMax)
    u = RCMax;
end
%dead zone and normalize
 if(u > RCMid + deadZone)
    y = (u-RCMid - deadZone)*k;
 elseif(u < RCMid - deadZone)
     y = (u - RCMid + deadZone)*k;
 else
     y = 0;
 end

 end

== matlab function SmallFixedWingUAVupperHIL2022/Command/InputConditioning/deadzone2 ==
function y = fcn(u)
%Function description:
%  Control the range of the remote control input from RCMin to RCMax, and set
%  a dead zone with a dead zone size of ±deadZone,the output y is
%  normalized to 0~1.You can get the RC calibration parameters in QGC.
RCMin = 1100;
RCMax = 1900;
RCMid = (RCMin + RCMax)/2;
deadZoneRate = 0.05;
deadZone = deadZoneRate*(RCMax - RCMin);
k = 1/(RCMax - RCMid - deadZone);
%Limiting
if(u < RCMin)
    u = RCMin;
elseif(u > RCMax)
    u = RCMax;
end
%dead zone and normalize
 if(u > RCMid + deadZone)
    y = (u-RCMid - deadZone)*k;
 elseif(u < RCMid - deadZone)
     y = (u - RCMid + deadZone)*k;
 else
     y = 0;
 end

 end
